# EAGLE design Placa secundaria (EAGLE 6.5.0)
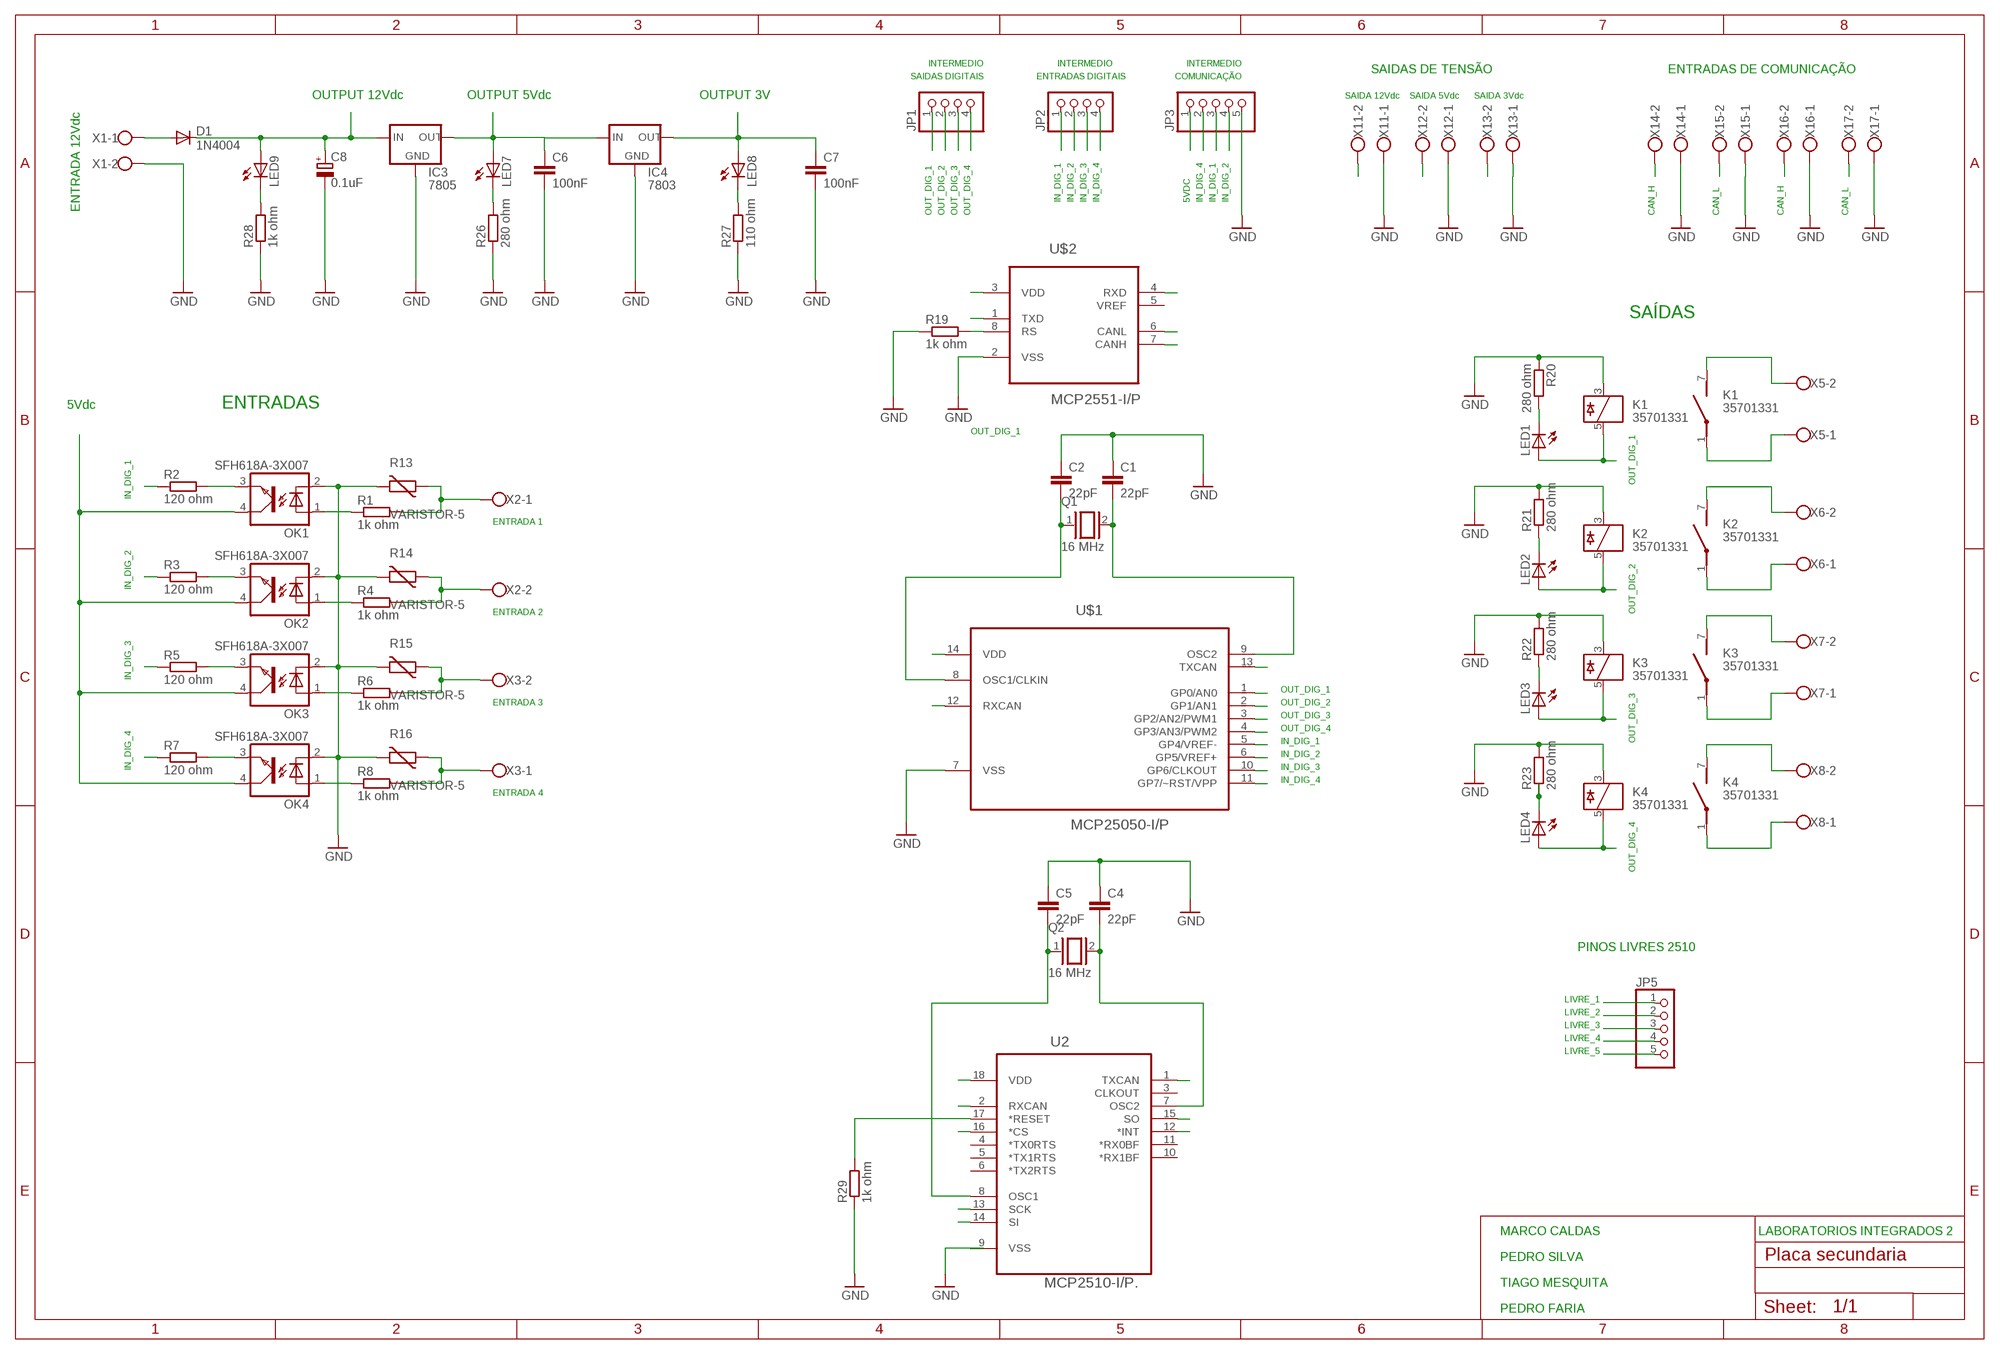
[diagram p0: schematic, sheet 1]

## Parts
C1  22pF  C-EU050-025X075  [C050-025X075]
C2  22pF  C-EU050-025X075  [C050-025X075]
C4  22pF  C-EU050-025X075  [C050-025X075]
C5  22pF  C-EU050-025X075  [C050-025X075]
C6  100nF  C-EU050-025X075  [C050-025X075]
C7  100nF  C-EU050-025X075  [C050-025X075]
C8  0.1uF  CPOL-EUE2.5-7  [E2,5-7]
D1  1N4004  [DO41-10]
IC3  7805  78XXS  [78XXS]
IC4  7803  78XXS  [78XXS]
JP1  PINHD-1X4  [1X04]
JP2  PINHD-1X4  [1X04]
JP3  PINHD-1X5/90  [1X05/90]
JP5  PINHD-1X5  [1X05]
K1  35701331  [REED]
K2  35701331  [REED]
K3  35701331  [REED]
K4  35701331  [REED]
LED1  LED5MM  [LED5MM]
LED2  LED5MM  [LED5MM]
LED3  LED5MM  [LED5MM]
LED4  LED5MM  [LED5MM]
LED7  LED5MM  [LED5MM]
LED8  LED5MM  [LED5MM]
LED9  LED5MM  [LED5MM]
OK1  SFH618A-3X007  [SMD4-7]
OK2  SFH618A-3X007  [SMD4-7]
OK3  SFH618A-3X007  [SMD4-7]
OK4  SFH618A-3X007  [SMD4-7]
Q1  16 MHz  XTAL/S  [QS]
Q2  16 MHz  XTAL/S  [QS]
R1  1k ohm  R-EU_0207/10  [0207/10]
R2  120 ohm  R-EU_0207/10  [0207/10]
R3  120 ohm  R-EU_0207/10  [0207/10]
R4  1k ohm  R-EU_0207/10  [0207/10]
R5  120 ohm  R-EU_0207/10  [0207/10]
R6  1k ohm  R-EU_0207/10  [0207/10]
R7  120 ohm  R-EU_0207/10  [0207/10]
R8  1k ohm  R-EU_0207/10  [0207/10]
R13  VARISTOR-5  [R-5]
R14  VARISTOR-5  [R-5]
R15  VARISTOR-5  [R-5]
R16  VARISTOR-5  [R-5]
R19  1k ohm  R-EU_0207/10  [0207/10]
R20  280 ohm  R-EU_0207/10  [0207/10]
R21  280 ohm  R-EU_0207/10  [0207/10]
R22  280 ohm  R-EU_0207/10  [0207/10]
R23  280 ohm  R-EU_0207/10  [0207/10]
R26  280 ohm  R-EU_0207/10  [0207/10]
R27  110 ohm  R-EU_0207/10  [0207/10]
R28  1k ohm  R-EU_0207/10  [0207/10]
R29  1k ohm  R-EU_0207/10  [0207/10]
U2  MCP2510-I/P.  [DIP254P762X533-18P]
U$1  MCP25050-I/P  [DIP254P762X432-14]
U$2  MCP2551-I/P  [DIP254P762X432-8]
X1  W237-102  [W237-102]
X2  W237-102  [W237-102]
X3  W237-102  [W237-102]
X5  W237-102  [W237-102]
X6  W237-102  [W237-102]
X7  W237-102  [W237-102]
X8  W237-102  [W237-102]
X11  W237-102  [W237-102]
X12  W237-102  [W237-102]
X13  W237-102  [W237-102]
X14  W237-102  [W237-102]
X15  W237-102  [W237-102]
X16  W237-102  [W237-102]
X17  W237-102  [W237-102]

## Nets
3VDC: C7.1 IC4.OUT LED8.A X13.2
5VDC: C6.1 IC3.OUT IC4.IN JP3.1 LED7.A OK1.4(COL) OK2.4(COL) OK3.4(COL) OK4.4(COL) U2.18(VDD) U$1.14(VDD) U$2.3(VDD) X12.2
12VDC: C8.+ D1.C IC3.IN LED9.A X11.2
CAN_H: U$2.7(CANH) X14.2 X16.2
CAN_L: U$2.6(CANL) X15.2 X17.2
CAN_RX: U2.1(TXCAN) U$1.13(TXCAN) U$2.4(RXD)
CAN_TX: U2.2(RXCAN) U$1.12(RXCAN) U$2.1(TXD)
GND: C1.1 C2.1 C4.1 C5.1 C6.2 C7.2 C8.- IC3.GND IC4.GND JP3.5 K1.3 K2.3 K3.3 K4.3 OK1.2(C) OK2.2(C) OK3.2(C) OK4.2(C) R13.2 R14.2 R15.2 R16.2 R19.1 R20.1 R21.2 R22.2 R23.2 R26.1 R27.1 R28.1 R29.1 U$1.7(VSS) U$2.2(VSS) X1.2 X11.1 X12.1 X14.1 X16.1 X17.1
IN_DIG_1: JP2.1 JP3.3 R2.1 U$1.5(GP4/VREF-)
IN_DIG_2: JP2.2 JP3.4 R3.1 U$1.6(GP5/VREF+)
IN_DIG_3: JP2.3 R5.1 U$1.10(GP6/CLKOUT)
IN_DIG_4: JP2.4 JP3.2 R7.1 U$1.11(GP7/~RST/VPP)
LIVRE_1: JP5.1 U2.16(*CS)
LIVRE_2: JP5.2 U2.13(SCK)
LIVRE_3: JP5.3 U2.14(SI)
LIVRE_4: JP1.3 JP5.4 K3.5 LED3.A U2.12(*INT) U$1.3(GP2/AN2/PWM1)
LIVRE_5: JP5.5 U2.15(SO)
N$1: OK1.3(EMIT) R2.2
N$2: OK1.1(A) R1.1
N$3: X15.1
N$4: K1.7(2:S) X5.2
N$5: OK2.1(A) R4.1
N$6: OK3.1(A) R6.1
N$7: OK4.1(A) R8.1
N$8: OK2.3(EMIT) R3.2
N$9: OK3.3(EMIT) R5.2
N$10: OK4.3(EMIT) R7.2
N$13: K1.1(2:P) X5.1
N$14: R1.2 R13.1 X2.1
N$16: C2.2 Q1.1 U$1.8(OSC1/CLKIN)
N$17: R4.2 R14.1 X2.2
N$18: R6.2 R15.1 X3.2
N$19: R8.2 R16.1 X3.1
N$22: LED2.K(C) R21.1
N$24: LED1.K(C) R20.2
N$27: K2.7(2:S) X6.2
N$30: LED3.K(C) R22.1
N$31: R19.2 U$2.8(RS)
N$32: D1.A X1.1
N$33: C4.2 Q2.2 U2.7(OSC2)
N$34: C5.2 Q2.1 U2.8(OSC1)
N$35: R29.2 U2.17(*RESET)
N$38: K2.1(2:P) X6.1
N$39: LED4.K(C) R23.1
N$41: K3.7(2:S) X7.2
N$43: LED7.K(C) R26.2
N$44: K3.1(2:P) X7.1
N$46: LED8.K(C) R27.2
N$47: K4.7(2:S) X8.2
N$48: LED9.K(C) R28.2
N$49: C1.2 Q1.2 U$1.9(OSC2)
N$50: K4.1(2:P) X8.1
N$57: X13.1
OUT_DIG_1: JP1.1 K1.5 LED1.A U$1.1(GP0/AN0)
OUT_DIG_2: JP1.2 K2.5 LED2.A U$1.2(GP1/AN1)
OUT_DIG_4: JP1.4 K4.5 LED4.A U$1.4(GP3/AN3/PWM2)
Unconnected: U2.3(CLKOUT) U2.4(*TX0RTS) U2.5(*TX1RTS) U2.6(*TX2RTS) U2.10(*RX1BF) U2.11(*RX0BF) U$2.5(VREF)

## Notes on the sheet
- INTERMEDIO | INTERMEDIO | INTERMEDIO
- SAIDAS DIGITAIS | ENTRADAS DIGITAIS | COMUNICAÇÃO | SAIDAS DE TENSÃO | ENTRADAS DE COMUNICAÇÃO
- OUTPUT 12Vdc | OUTPUT 5Vdc | OUTPUT 3V | SAIDA 12Vdc | SAIDA 5Vdc | SAIDA 3Vdc
- IN_DIG_1 | IN_DIG_2 | IN_DIG_3 | IN_DIG_4 | 5VDC | IN_DIG_4 | IN_DIG_1 | IN_DIG_2
- ENTRADA 12Vdc | OUT_DIG_1 | OUT_DIG_2 | OUT_DIG_3 | OUT_DIG_4 | CAN_H | CAN_L | CAN_H | CAN_L
- SAÍDAS
- 5Vdc | ENTRADAS
- OUT_DIG_1 | OUT_DIG_1
- IN_DIG_1
- ENTRADA 1
- OUT_DIG_2
- IN_DIG_2
- ENTRADA 2
- IN_DIG_3
- OUT_DIG_1 | OUT_DIG_3
- ENTRADA 3 | OUT_DIG_2
- OUT_DIG_3
- OUT_DIG_4
- IN_DIG_1
- IN_DIG_2
- IN_DIG_4 | IN_DIG_3
- IN_DIG_4
- ENTRADA 4
- OUT_DIG_4
- PINOS LIVRES 2510
- LIVRE_1
- LIVRE_2
- LIVRE_3
- LIVRE_4
- LIVRE_5
- MARCO CALDAS | LABORATORIOS INTEGRADOS 2
- PEDRO SILVA
- TIAGO MESQUITA
- PEDRO FARIA

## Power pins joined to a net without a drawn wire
VSS: U2.9(VSS)

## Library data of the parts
C1 C2 C4-C7 = rcl:C-EU: CAPACITOR, European symbol
C8 = rcl:CPOL-EU: POLARIZED CAPACITOR, European symbol
D1 = diode:1N4004: DIODE
IC3 IC4 = v-reg:78XXS: VOLTAGE REGULATOR
JP1 JP2 = pinhead:PINHD-1X4: PIN HEADER
JP3 JP5 = pinhead:PINHD-1X5: PIN HEADER
K1-K4 = relay:35701331: RELAY reed, 1 x norm. open with polarity; OC_FARNELL: unknown; OC_NEWARK: unknown
LED1-LED4 LED7-LED9 = led:LED: LED
OK1-OK4 = optocoupler:SFH618?*: Optocoupler, Phototransistor Output, Low Input Current Source: Data sheet; OC_FARNELL: unknown; OC_NEWARK: unknown
Q1 Q2 = special:XTAL/S: CRYSTAL
R1-R8 R19-R23 R26-R29 = rcl:R-EU_: RESISTOR, European symbol
R13-R16 = varistor:VARISTOR: VARISTOR
U2 = MCP2510:MCP2510-I/P.: IC, Stand-Alone CAN Controller with SPI Interface, DIP-18; MPN: MCP2510-I/P.; OC_FARNELL: 9758534; OC_NEWARK: 12C1807; PACKAGE: DIP-18; SUPPLIER: Microchip
U$1 = mcp25050:MCP25050-I/P: CAN I/O Expander Family; MPN: MCP25050-I/P; OC_FARNELL: 1439736; OC_NEWARK: 59K0224; PACKAGE: DIP-14; SUPPLIER: Microchip
U$2 = MCP:MCP2551-I/P: High-Speed CAN Transceiver; DESCRIPTION: CAN CTRL; MPN: MCP2551-I/P; OC_FARNELL: 1292240; OC_NEWARK: 61K2947; PACKAGE: PDIP-8; SUPPLIER: Microchip
X1-X3 X5-X8 X11-X17 = con-wago-500:W237-102: WAGO SCREW CLAMP; MPN: 237-102; OC_FARNELL: unknown; OC_NEWARK: 70K9898

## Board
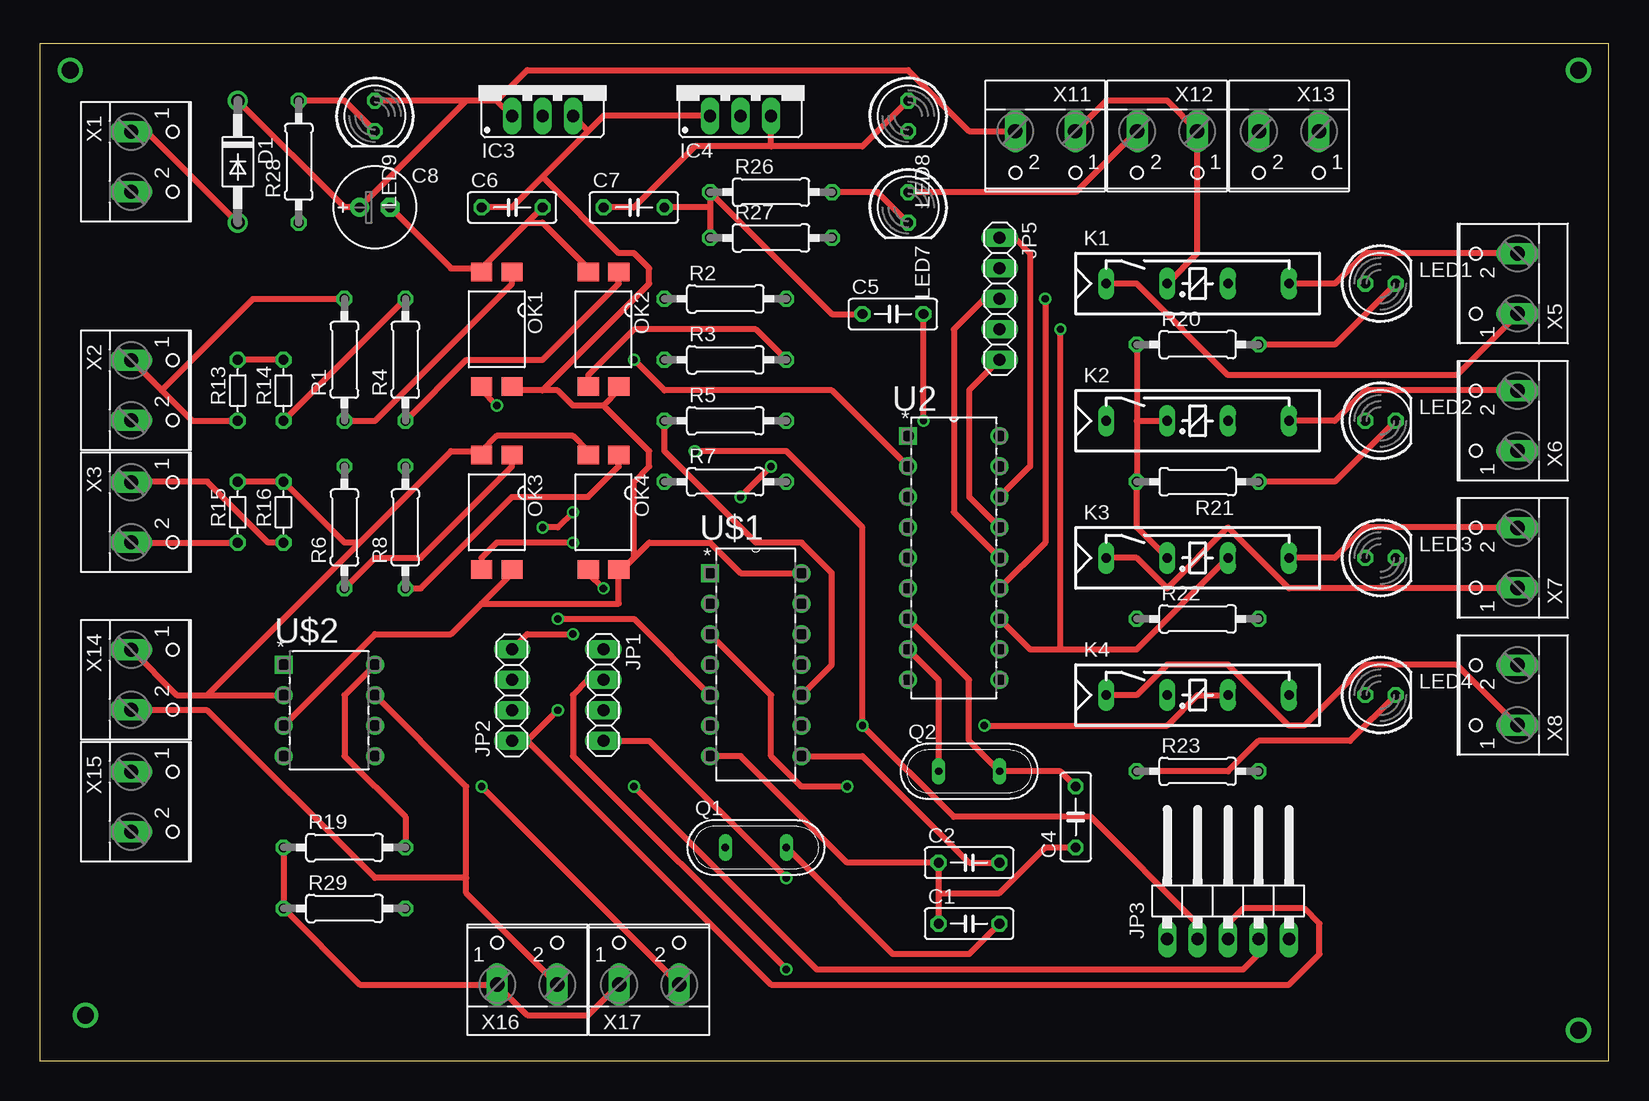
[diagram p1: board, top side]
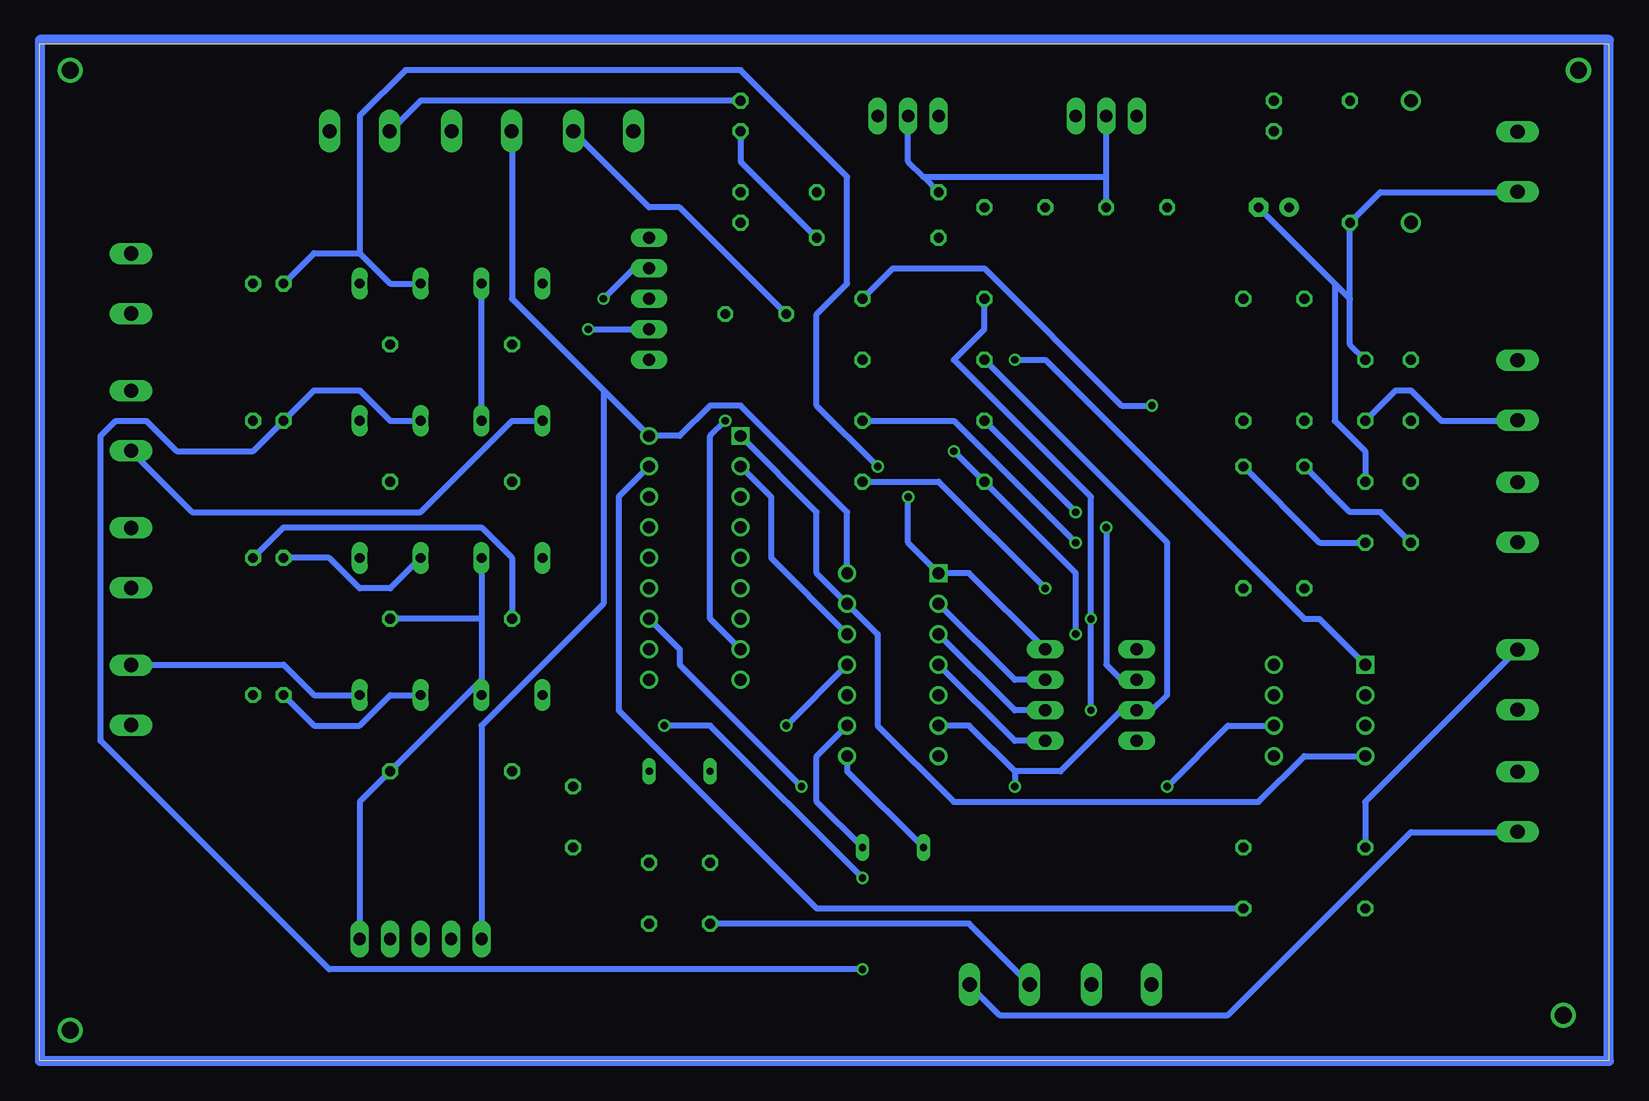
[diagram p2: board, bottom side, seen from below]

Size 130.79 x 84.76 mm. Coordinates in mm from the lower left corner, seen from the top.
Outline: 0,0 130.79,0 130.79,84.76 0,84.76 0,0
Copper layers (1*16): Top 0.035mm / dielectric 1.5mm / Bottom 0.035mm
Design rules "default *": minimum track width 20mil, minimum drill 24mil, track to track 16mil, track to pad 16mil, pad to pad 8mil, via to via 16mil, smd to smd 8mil, copper to edge 40mil, drill to drill 8mil, minimum pad ring 10mil, minimum via ring 8mil, stop-mask expansion 4mil, vias tented up to drill 0mil, thermal gap 15mil

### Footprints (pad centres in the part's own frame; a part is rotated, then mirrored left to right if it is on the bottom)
C050-025X075 = drill 0.813 octagon: 1 -2.54,0; 2 2.54,0
E2,5-7 = drill 0.813 pad 1.6: + -1.27,0 | drill 0.813 pad 1.6 octagon: - 1.27,0
DO41-10 = drill 1.118: A 5.08,0; C -5.08,0
78XXS = drill 1.016 long: GND 0,-2.54; IN -2.54,-2.54; OUT 2.54,-2.54
1X04 = drill 1.016 long: 1 -3.81,0; 2 -1.27,0; 3 1.27,0; 4 3.81,0
1X05/90 = drill 1.016 long: 1 -5.08,-3.81; 2 -2.54,-3.81; 3 0,-3.81; 4 2.54,-3.81; 5 5.08,-3.81
1X05 = drill 1.016 long: 1 -5.08,0; 2 -2.54,0; 3 0,0; 4 2.54,0; 5 5.08,0
REED = drill 0.813 long: 1 -17.78,2.54; 3 -12.7,2.54; 5 -7.62,2.54; 7 -2.54,2.54
LED5MM = drill 0.813 octagon: A -1.27,0; K 1.27,0
SMD4-7 = smd 1.78 x 1.55: 1 -1.27,-4.77; 2 1.27,-4.77; 3 1.27,4.77; 4 -1.27,4.77
QS = drill 0.61 long: 1 -2.54,0; 2 2.54,0
0207/10 = drill 0.813 octagon: 1 -5.08,0; 2 5.08,0
R-5 = drill 0.813 octagon: 1 -2.54,0; 2 2.54,0
DIP254P762X533-18P = drill 0.991 square: 1 -7.62,20.32 | drill 0.991: 2 -7.62,17.78; 3 -7.62,15.24; 4 -7.62,12.7; 5 -7.62,10.16; 6 -7.62,7.62; 7 -7.62,5.08; 8 -7.62,2.54; 9 -7.62,0; 10 0,0; 11 0,2.54; 12 0,5.08; 13 0,7.62; 14 0,10.16; 15 0,12.7; 16 0,15.24; 17 0,17.78; 18 0,20.32
DIP254P762X432-14 = drill 0.991 square: 1 -7.62,15.24 | drill 0.991: 2 -7.62,12.7; 3 -7.62,10.16; 4 -7.62,7.62; 5 -7.62,5.08; 6 -7.62,2.54; 7 -7.62,0; 8 0,0; 9 0,2.54; 10 0,5.08; 11 0,7.62; 12 0,10.16; 13 0,12.7; 14 0,15.24
DIP254P762X432-8 = drill 0.991 square: 1 -7.62,7.62 | drill 0.991: 2 -7.62,5.08; 3 -7.62,2.54; 4 -7.62,0; 5 0,0; 6 0,2.54; 7 0,5.08; 8 0,7.62
W237-102 = drill 1.194 long: 1 -2.5,-1.27; 2 2.5,-1.27

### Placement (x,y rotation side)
C1  77.47,11.43 0 top
C2  77.47,16.51 0 top
C4  86.36,20.32 90 top
C5  71.12,62.23 0 top
C6  39.37,71.12 0 top
C7  49.53,71.12 0 top
C8  27.94,71.12 0 top
D1  16.51,74.93 270 top
IC3  41.91,81.28 0 top
IC4  58.42,81.28 0 top
JP1  46.99,30.48 270 top
JP2  39.37,30.48 90 top
JP3  99.06,13.97 0 top
JP5  80.01,63.5 270 top
K1  106.68,62.23 0 top
K2  106.68,50.8 0 top
K3  106.68,39.37 0 top
K4  106.68,27.94 0 top
LED1  111.76,64.77 0 top
LED2  111.76,53.34 0 top
LED3  111.76,41.91 0 top
LED4  111.76,30.48 0 top
LED7  72.39,71.12 270 top
LED8  72.39,78.74 270 top
LED9  27.94,78.74 270 top
OK1  38.1,60.96 180 top
OK2  46.99,60.96 180 top
OK3  38.1,45.72 180 top
OK4  46.99,45.72 180 top
Q1  59.69,17.78 0 top
Q2  77.47,24.13 0 top
R1  25.4,58.42 90 top
R2  57.15,63.5 0 top
R3  57.15,58.42 0 top
R4  30.48,58.42 90 top
R5  57.15,53.34 0 top
R6  25.4,44.45 90 top
R7  57.15,48.26 0 top
R8  30.48,44.45 90 top
R13  16.51,55.88 90 top
R14  20.32,55.88 90 top
R15  16.51,45.72 90 top
R16  20.32,45.72 90 top
R19  25.4,17.78 0 top
R20  96.52,59.69 0 top
R21  96.52,48.26 180 top
R22  96.52,36.83 0 top
R23  96.52,24.13 0 top
R26  60.96,72.39 0 top
R27  60.96,68.58 0 top
R28  21.59,74.93 90 top
R29  25.4,12.7 0 top
U2  80.01,31.75 0 top
U$1  63.5,25.4 0 top
U$2  27.94,25.4 0 top
X1  8.89,74.93 270 top
X2  8.89,55.88 270 top
X3  8.89,45.72 270 top
X5  121.92,64.77 90 top
X6  121.92,53.34 90 top
X7  121.92,41.91 90 top
X8  121.92,30.48 90 top
X11  83.82,76.2 180 top
X12  93.98,76.2 180 top
X13  104.14,76.2 180 top
X14  8.89,31.75 270 top
X15  8.89,21.59 270 top
X16  40.64,7.62 0 top
X17  50.8,7.62 0 top

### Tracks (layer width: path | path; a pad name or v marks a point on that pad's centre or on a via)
3VDC
  Top 0.508: C7.1 49.53,71.12 54.61,76.2 60.96,76.2 | 60.96,76.2 68.58,76.2 LED8.A | 60.96,76.2 IC4.OUT
  Bottom 0.508: LED8.A 99.06,80.01 101.6,77.47 X13.2
5VDC
  Top 0.508: LED7.A 86.36,72.39 91.44,77.47 X12.2 | C6.1 39.37,71.12 41.91,73.66 | 45.72,77.47 46.99,78.74 IC4.IN | 45.72,77.47 41.91,73.66 | 45.72,77.47 IC3.OUT | 41.91,55.88 43.18,55.88 44.45,54.61 46.99,54.61 | 41.91,55.88 39.37,55.88 OK1.4 | 46.99,54.61 48.26,55.88 OK2.4 | 36.83,38.1 34.29,35.56 27.94,35.56 U$2.3 | 36.83,38.1 39.37,40.64 OK3.4 | 48.26,40.64 48.26,38.1 36.83,38.1 | U$1.14 58.42,40.64 55.88,43.18 50.8,43.18 49.53,41.91 | 48.26,40.64 49.53,41.91 | 48.26,40.64 OK4.4 | 46.99,54.61 50.8,50.8 50.8,49.53 49.53,48.26 49.53,41.91 | 41.91,73.66 48.26,67.31 49.53,67.31 50.8,66.04 50.8,64.77 41.91,55.88
  Bottom 0.508: 83.82,55.88 91.44,63.5 91.44,77.47 X12.2 | 83.82,55.88 U2.18 77.47,52.07 74.93,54.61 72.39,54.61 63.5,45.72 U$1.14 | JP3.1 93.98,27.94 83.82,38.1 83.82,55.88
12VDC
  Top 0.508: 38.1,80.01 35.56,80.01 | 35.56,80.01 LED9.A | IC3.IN 38.1,80.01 | 35.56,80.01 C8.+ 25.4,71.12 D1.C | X11.2 77.47,77.47 72.39,82.55 40.64,82.55 38.1,80.01
CAN_H
  Top 0.508: U$2.7 35.56,22.86 35.56,15.24 | 35.56,15.24 35.56,13.97 43.18,6.35 X16.2 | 35.56,15.24 27.94,15.24 13.97,29.21 7.62,29.21 X14.2
CAN_L  (via drill 0.61)
  Top 0.508: v36.83,22.86 53.34,6.35 X17.2
  Bottom 0.508: U$2.6 31.75,27.94 v36.83,22.86 | X15.2 7.62,19.05 16.51,19.05 31.75,3.81 50.8,3.81 53.34,6.35 X17.2
CAN_RX
  Bottom 0.508: U$2.4 25.4,25.4 29.21,21.59 54.61,21.59 60.96,27.94 60.96,35.56 U$1.13 66.04,40.64 66.04,45.72 U2.1
CAN_TX  (via drill 0.61)
  Top 0.508: v49.53,58.42 52.07,55.88 66.04,55.88 U2.2
  Bottom 0.508: U$2.1 24.13,36.83 25.4,36.83 46.99,58.42 v49.53,58.42 | U$1.12 69.85,41.91 69.85,46.99 U2.2
GND
  Top 0.508: 96.52,77.47 93.98,80.01 88.9,80.01 86.36,77.47 X11.1 | R20.1 91.44,53.34 | 91.44,53.34 R21.2 91.44,44.45 K3.3 | 91.44,53.34 K2.3 | 96.52,77.47 96.52,67.31 K1.3 | 96.52,77.47 X12.1 | C6.2 40.64,69.85 | 40.64,69.85 36.83,66.04 | 40.64,69.85 41.91,69.85 45.72,66.04 OK2.2 | 55.88,71.12 R26.1 66.04,62.23 C5.1 | 55.88,71.12 R27.1 | 55.88,71.12 C7.2 | R15.2 R16.2 25.4,43.18 26.67,43.18 | R14.2 R13.2 | 74.93,13.97 C2.1 67.31,16.51 58.42,25.4 U$1.7 | 74.93,13.97 C1.1 | C4.1 83.82,17.78 80.01,13.97 74.93,13.97 | R19.1 R29.1 26.67,6.35 38.1,6.35 | 38.1,6.35 40.64,3.81 45.72,3.81 48.26,6.35 X17.1 | 38.1,6.35 X16.1 | 36.83,50.8 38.1,52.07 44.45,52.07 45.72,50.8 OK4.2 | 13.97,30.48 11.43,30.48 7.62,34.29 X14.1 | 13.97,30.48 U$2.2 | 36.83,50.8 34.29,50.8 26.67,43.18 | 13.97,30.48 26.67,43.18 | 36.83,50.8 OK3.2 | 36.83,66.04 34.29,66.04 C8.- | 36.83,66.04 OK1.2
  Bottom 0.508: K2.3 K1.3 | K3.3 93.98,36.83 | 93.98,36.83 93.98,31.75 | 93.98,31.75 R23.2 104.14,21.59 JP3.5 | 93.98,31.75 K4.3 | 93.98,36.83 R22.2 | C6.2 41.91,73.66 | 41.91,73.66 IC3.GND | IC4.GND 58.42,74.93 57.15,73.66 | R26.1 57.15,73.66 | 57.15,73.66 41.91,73.66 | 21.59,63.5 21.59,59.69 R14.2 | 21.59,63.5 R28.1 19.05,72.39 7.62,72.39 X1.2 | 21.59,63.5 22.86,64.77 | 22.86,64.77 C8.- | R16.2 20.32,50.8 22.86,53.34 22.86,64.77 | R19.1 20.32,21.59 7.62,34.29 X14.1 | C1.1 53.34,11.43 48.26,6.35 X17.1 | C5.1 77.47,71.12 80.01,71.12 86.36,77.47 X11.1
IN_DIG_1  (via drill 0.61)
  Top 0.508: 40.64,26.67 v43.18,29.21 | U$1.5 49.53,36.83 v43.18,36.83 | JP3.3 99.06,11.43 100.33,12.7 105.41,12.7 106.68,11.43 106.68,8.89 104.14,6.35 60.96,6.35 40.64,26.67 | 40.64,26.67 JP2.1
  Bottom 0.508: R2.1 52.07,60.96 54.61,58.42 43.18,46.99 v43.18,36.83 v43.18,29.21
IN_DIG_2  (via drill 0.61)
  Top 0.508: JP3.4 101.6,8.89 100.33,7.62 64.77,7.62 v49.53,22.86
  Bottom 0.508: R3.1 36.83,43.18 36.83,30.48 38.1,29.21 JP2.2 40.64,29.21 45.72,24.13 49.53,24.13 | U$1.6 53.34,27.94 49.53,24.13 | 49.53,24.13 v49.53,22.86
IN_DIG_3  (via drill 0.61)
  Top 0.508: R5.1 52.07,50.8 59.69,43.18 63.5,43.18 66.04,40.64 66.04,33.02 U$1.10 | v41.91,44.45 43.18,44.45 v44.45,45.72
  Bottom 0.508: JP2.3 40.64,31.75 41.91,33.02 v41.91,44.45 | R5.1 v44.45,45.72
IN_DIG_4  (via drill 0.61)
  Top 0.508: v44.45,35.56 40.64,35.56 JP2.4 | JP3.2 96.52,11.43 87.63,20.32 76.2,20.32 v68.58,27.94 68.58,44.45 62.23,50.8 v54.61,50.8
  Bottom 0.508: v44.45,35.56 44.45,40.64 R7.1 v54.61,50.8 | v68.58,27.94 U$1.11
LIVRE_1
  Top 0.508: U2.16 82.55,49.53 82.55,67.31 81.28,68.58 JP5.1
LIVRE_2  (via drill 0.61)
  Top 0.508: U2.13 83.82,43.18 v83.82,63.5
  Bottom 0.508: v83.82,63.5 81.28,66.04 JP5.2
LIVRE_3
  Top 0.508: U2.14 76.2,45.72 76.2,60.96 78.74,63.5 JP5.3
LIVRE_4  (via drill 0.61)
  Top 0.508: K3.5 91.44,34.29 85.09,34.29 | 85.09,34.29 82.55,34.29 U2.12 | 85.09,34.29 v85.09,60.96 | U$1.3 60.96,30.48 60.96,25.4 63.5,22.86 v67.31,22.86
  Bottom 0.508: U$1.3 49.53,29.21 JP1.3 | LED3.A 106.68,41.91 104.14,39.37 101.6,39.37 K3.5 | v85.09,60.96 JP5.4 | v67.31,22.86 77.47,33.02 77.47,34.29 U2.12
LIVRE_5
  Top 0.508: U2.15 77.47,46.99 77.47,55.88 JP5.5
N$1  (via drill 0.61)
  Top 0.508: v38.1,54.61 36.83,55.88 OK1.3
  Bottom 0.508: v38.1,54.61 40.64,54.61 52.07,66.04 59.69,66.04 R2.2
N$2
  Top 0.508: R1.1 27.94,53.34 39.37,64.77 OK1.1 39.37,66.04
N$4
  Top 0.508: K1.7 107.95,64.77 110.49,67.31 123.19,67.31 X5.2
N$5
  Top 0.508: R4.1 35.56,58.42 41.91,58.42 48.26,64.77 OK2.1 48.26,66.04
N$6
  Top 0.508: R6.1 27.94,41.91 31.75,41.91 39.37,49.53 OK3.1 39.37,50.8
N$7
  Top 0.508: R8.1 31.75,39.37 39.37,46.99 45.72,46.99 48.26,49.53 OK4.1 48.26,50.8
N$8
  Top 0.508: R3.2 59.69,60.96 49.53,60.96 45.72,57.15 OK2.3 45.72,55.88
N$9  (via drill 0.61)
  Top 0.508: v44.45,43.18 38.1,43.18 36.83,41.91 OK3.3 36.83,40.64
  Bottom 0.508: v44.45,43.18 54.61,53.34 R5.2
N$10  (via drill 0.61)
  Top 0.508: v46.99,39.37 45.72,40.64 OK4.3
  Bottom 0.508: v46.99,39.37 55.88,48.26 R7.2
N$11
  Bottom 0.813: 0,85.09 130.81,85.09 130.81,0 0,0 0,85.09
N$12  (via drill 1.4)
  other vias: 2.54,82.55
N$13
  Top 0.508: K1.1 91.44,64.77 99.06,57.15 118.11,57.15 123.19,62.23 X5.1
N$14
  Top 0.508: R13.1 12.7,53.34 10.16,55.88 | 10.16,55.88 7.62,58.42 X2.1 | R1.2 17.78,63.5 10.16,55.88
N$15  (via drill 1.4)
  other vias: 128.27,82.55
N$16
  Top 0.508: C2.2 77.47,16.51 68.58,25.4 U$1.8
  Bottom 0.508: Q1.1 63.5,24.13 U$1.8
N$17
  Top 0.508: R4.2 R14.1
  Bottom 0.508: R14.1 17.78,55.88 16.51,55.88 13.97,53.34 7.62,53.34 X2.2
N$18
  Top 0.508: R15.1 7.62,43.18 X3.2
  Bottom 0.508: R6.2 21.59,45.72 19.05,45.72 R15.1
N$19
  Top 0.508: R16.1 19.05,43.18 13.97,48.26 7.62,48.26 X3.1
  Bottom 0.508: R16.1 24.13,43.18 R8.2
N$20  (via drill 1.4)
  other vias: 128.27,2.54
N$21  (via drill 1.4)
  other vias: 3.81,3.81
N$22
  Top 0.508: R21.1 107.95,48.26 LED2.K
N$24
  Top 0.508: R20.2 107.95,59.69 LED1.K
N$27
  Top 0.508: K2.7 107.95,53.34 110.49,55.88 123.19,55.88 X6.2
N$30
  Bottom 0.508: R22.1 91.44,41.91 93.98,44.45 110.49,44.45 LED3.K
N$31
  Top 0.508: R19.2 30.48,20.32 25.4,25.4 25.4,30.48 U$2.8
N$32
  Top 0.508: D1.A 8.89,77.47 7.62,77.47 X1.1
N$33
  Top 0.508: C4.2 85.09,24.13 Q2.2 77.47,26.67 77.47,31.75 U2.7
N$34  (via drill 0.61)
  Top 0.508: Q2.1 74.93,31.75 U2.8 | v73.66,53.34 C5.2
  Bottom 0.508: v73.66,53.34 74.93,52.07 74.93,36.83 U2.8
N$35
  Bottom 0.508: R29.2 66.04,12.7 82.55,29.21 82.55,46.99 U2.17
N$38
  Bottom 0.508: K2.1 91.44,53.34 99.06,45.72 118.11,45.72 123.19,50.8 X6.1
N$39
  Top 0.508: R23.1 99.06,24.13 101.6,26.67 109.22,26.67 LED4.K
N$41
  Top 0.508: K3.7 107.95,41.91 110.49,44.45 123.19,44.45 X7.2
N$43
  Top 0.508: R26.2 69.85,72.39 LED7.K
N$44
  Top 0.508: K3.1 91.44,41.91 93.98,39.37 99.06,44.45 104.14,39.37 123.19,39.37 X7.1
N$46
  Bottom 0.508: R27.2 72.39,74.93 LED8.K
N$47
  Bottom 0.508: K4.7 107.95,30.48 110.49,33.02 123.19,33.02 X8.2
N$48
  Top 0.508: R28.2 25.4,80.01 LED9.K
N$49
  Top 0.508: Q1.2 71.12,8.89 77.47,8.89 C1.2
  Bottom 0.508: U$1.9 66.04,25.4 66.04,21.59 Q1.2
N$50
  Top 0.508: K4.1 91.44,30.48 93.98,33.02 99.06,33.02 104.14,27.94 105.41,27.94 110.49,33.02 118.11,33.02 123.19,27.94 X8.1
OUT_DIG_1  (via drill 0.61)
  Top 0.508: v58.42,46.99 v60.96,49.53
  Bottom 0.508: K1.5 101.6,64.77 104.14,67.31 | 104.14,67.31 107.95,67.31 LED1.A | JP1.1 53.34,40.64 U$1.1 58.42,43.18 v58.42,46.99 | 104.14,67.31 104.14,78.74 100.33,82.55 72.39,82.55 63.5,73.66 63.5,64.77 66.04,62.23 66.04,54.61 v60.96,49.53
OUT_DIG_2  (via drill 0.61)
  Top 0.508: v62.23,7.62 44.45,25.4 44.45,30.48 45.72,31.75 JP1.2
  Bottom 0.508: K2.5 101.6,53.34 104.14,55.88 107.95,55.88 LED2.A 113.03,50.8 119.38,50.8 121.92,53.34 124.46,53.34 125.73,52.07 125.73,26.67 106.68,7.62 v62.23,7.62 | U$1.2 49.53,31.75 JP1.2
OUT_DIG_4  (via drill 0.61)
  Top 0.508: K4.5 96.52,30.48 93.98,27.94 v78.74,27.94 | v62.23,15.24 50.8,26.67 JP1.4
  Bottom 0.508: K4.5 101.6,30.48 104.14,27.94 107.95,27.94 LED4.A | U$1.4 49.53,26.67 JP1.4 | v78.74,27.94 74.93,27.94 v62.23,15.24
